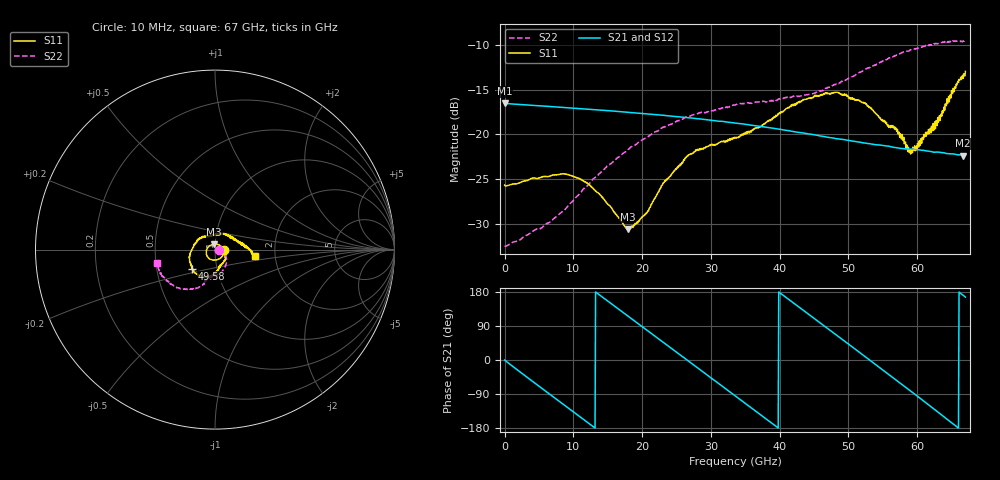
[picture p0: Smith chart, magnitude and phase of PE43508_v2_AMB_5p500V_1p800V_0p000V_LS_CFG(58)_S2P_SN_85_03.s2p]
!Keysight Technologies,N5227A,US51270237,A.10.43.00
!Date: Wednesday, August 22, 2018 17:12:39
!Correction: S11(Full 2 Port(1,3))
!S31(Full 2 Port(1,3))
!S13(Full 2 Port(1,3))
!S33(Full 2 Port(1,3))
!S2P File: Measurements: S11, S31, S13, S33:
# Hz S  dB  R 50
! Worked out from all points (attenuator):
!   801 points, 10 MHz to 67 GHz, reference 50 ohm
!   highest |S21| = -16.53 dB at 10 MHz (marker M1); lowest = -22.4 dB at 66.67 GHz (marker M2)
!   lowest |S11| = -30.6 dB at 17.93 GHz (marker M3), VSWR 1.06, Z = 49.4 + j2.89 ohm
!   |S11| at or under -10 dB: start of sweep to end of sweep
!   |S22| runs from -32.5 to -9.5 dB; largest |S21 - S12| = 0.00073
!   S11 on the Smith chart (normalised r, x): 10 MHz: 1.11, -0.00; 49.58 GHz: 0.76, -0.17; 67 GHz: 1.56, -0.12
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1e7  -25.68 -0.7  -16.53 -0.2  -16.53 -0.2  -32.47 -0.5
2.522125e9  -25.30 -38.3  -16.68 -35.2  -16.68 -35.2  -31.63 -2.1
5.787888e9  -24.73 -81.7  -16.84 -79.8  -16.85 -79.8  -30.17 -4.7
8.7187e9  -24.42 -117.7  -17.00 -119.5  -17.00 -119.5  -28.47 -9.5
1.123082e10  -25.09 -146.9  -17.13 -153.5  -17.14 -153.5  -26.34 -15.9
1.441285e10  -27.22 171.5  -17.31 163.5  -17.31 163.5  -23.94 -25.9
1.792982e10  -30.59 99.4  -17.52 116.1  -17.52 116.1  -21.72 -39.0
2.060942e10  -28.77 37.5  -17.71 79.9  -17.71 79.9  -20.38 -48.6
2.236791e10  -26.44 4.9  -17.83 56.2  -17.82 56.2  -19.56 -55.6
2.6806e10  -22.31 -41.4  -18.15 -3.7  -18.15 -3.6  -18.00 -70.7
3.040671e10  -21.23 -62.5  -18.45 -52.4  -18.45 -52.3  -17.33 -81.5
3.3505e10  -20.37 -74.1  -18.73 -94.3  -18.73 -94.3  -16.70 -89.8
3.911541e10  -18.21 -86.2  -19.32 -170.2  -19.32 -170.1  -16.28 -99.3
4.472582e10  -15.89 -110.9  -20.00 113.6  -19.99 113.7  -15.48 -105.3
4.95826e10  -15.57 -139.4  -20.61 47.6  -20.60 47.6  -13.93 -108.1
5.251341e10  -16.62 -164.1  -20.98 7.7  -20.97 7.6  -12.68 -113.8
5.586291e10  -19.22 157.0  -21.32 -38.3  -21.31 -38.6  -11.48 -123.6
5.870999e10  -21.44 115.2  -21.64 -77.0  -21.65 -77.1  -10.68 -133.0
5.937989e10  -21.42 97.0  -21.66 -86.3  -21.68 -86.5  -10.46 -135.1
6.29806e10  -18.12 33.1  -21.97 -136.8  -22.00 -137.2  -9.87 -149.6
6.666505e10  -13.75 -6.5  -22.36 170.8  -22.43 170.9  -9.56 -164.7
6.7e10  -12.97 -9.4  -22.35 165.9  -22.42 166.0  -9.54 -166.6
